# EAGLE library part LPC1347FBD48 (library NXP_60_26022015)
32-bit ARM Cortex-M3 microcontroller; up to 64 kB flash; up to 12 kB SRAM; USB device; USART; EEPROM The LPC1315/16/17/45/46/47 are ARM Cortex-M3 based microcontrollers for embedded applications featuring a high level of integration and low power consumption. The ARM Cortex-M3 is a next generation core that offers system enhancements such as enhanced debug features and a higher level of support block integration. The LPC1315/16/17/45/46/47 operate at CPU frequencies of up to 72 MHz. The ARM Cortex-M3 CPU incorporates a 3-stage pipeline and uses a Harvard architecture with separate local instruction and data buses as well as a third bus for peripherals. The ARM Cortex-M3 CPU also includes an internal prefetch unit that supports speculative branching. Equipped with a highly flexible and configurable Full-Speed USB 2.0 device controller available on the LPC1345/46/47, this series brings unparalleled design flexibility and seamless integration to today’s demanding connectivity solutions. The peripheral complement of the LPC1315/16/17/45/46/47 includes up to 64 kB of flash memory, 8 kB or 10 kB of SRAM data memory, one Fast-mode Plus I 2 C-bus interface, one RS-485/EIA-485 USART with support for synchronous mode and smart card interface, two SSP interfaces, four general purpose counter/timers, an 8-channel, 12-bit ADC, and up to 51 general purpose I/O pins. AAL Eindhoven MK
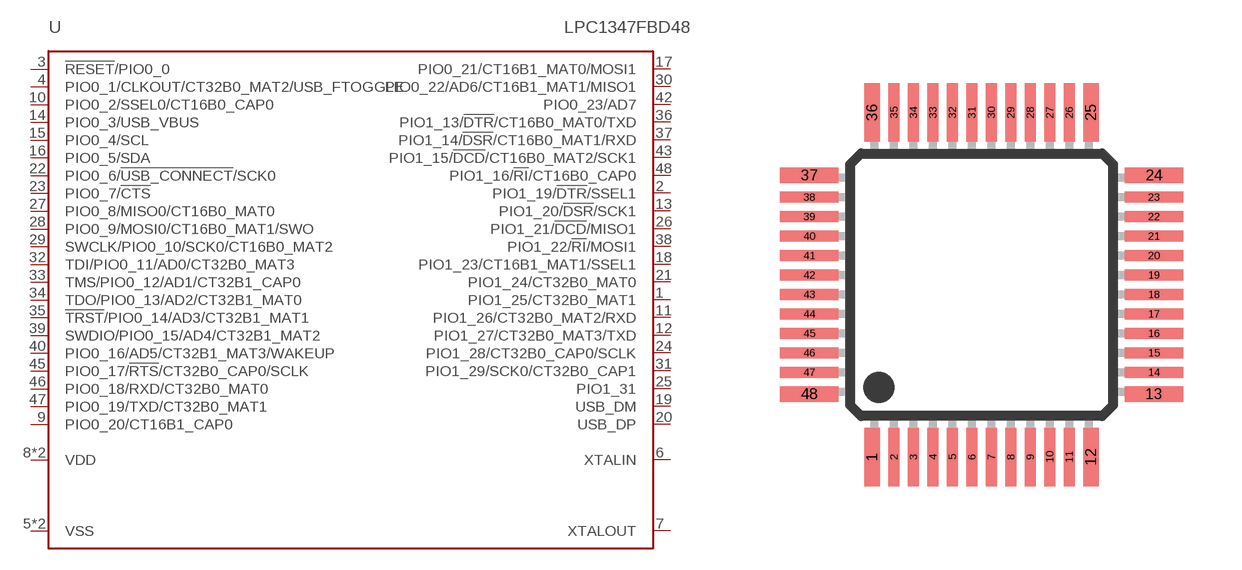
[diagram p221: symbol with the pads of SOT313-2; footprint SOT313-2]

Designator prefix U

## LPC1347FBD48 (EEPROM: 4kB; FLASH: 64kB; GPIO: 40; SRAM0: 8kB; SRAM1: 2kB; SRAM_USB: 2kB; USB: yes)  [SOT313-2]
1  PIO1_25/CT32B0_MAT1
2  PIO1_19/!DTR!/SSEL1
3  !RESET!/PIO0_0
4  PIO0_1/CLKOUT/CT32B0_MAT2/USB_FTOGGLE
5  VSS  pwr
6  XTALIN  in
7  XTALOUT  out
8  VDD  pwr
9  PIO0_20/CT16B1_CAP0
10  PIO0_2/SSEL0/CT16B0_CAP0
11  PIO1_26/CT32B0_MAT2/RXD
12  PIO1_27/CT32B0_MAT3/TXD
13  PIO1_20/!DSR!/SCK1
14  PIO0_3/USB_VBUS
15  PIO0_4/SCL
16  PIO0_5/SDA
17  PIO0_21/CT16B1_MAT0/MOSI1
18  PIO1_23/CT16B1_MAT1/SSEL1
19  USB_DM
20  USB_DP
21  PIO1_24/CT32B0_MAT0
22  PIO0_6/!USB_CONNECT!/SCK0
23  PIO0_7/!CTS!
24  PIO1_28/CT32B0_CAP0/SCLK
25  PIO1_31
26  PIO1_21/!DCD!/MISO1
27  PIO0_8/MISO0/CT16B0_MAT0
28  PIO0_9/MOSI0/CT16B0_MAT1/SWO
29  SWCLK/PIO0_10/SCK0/CT16B0_MAT2
30  PIO0_22/AD6/CT16B1_MAT1/MISO1
31  PIO1_29/SCK0/CT32B0_CAP1
32  TDI/PIO0_11/AD0/CT32B0_MAT3
33  TMS/PIO0_12/AD1/CT32B1_CAP0
34  TDO/PIO0_13/AD2/CT32B1_MAT0
35  !TRST!/PIO0_14/AD3/CT32B1_MAT1
36  PIO1_13/!DTR!/CT16B0_MAT0/TXD
37  PIO1_14/!DSR!/CT16B0_MAT1/RXD
38  PIO1_22/!RI!/MOSI1
39  SWDIO/PIO0_15/AD4/CT32B1_MAT2
40  PIO0_16/AD5/CT32B1_MAT3/WAKEUP
41  VSS  pwr
42  PIO0_23/AD7
43  PIO1_15/!DCD!/CT16B0_MAT2/SCK1
44  VDD  pwr
45  PIO0_17/!RTS!/CT32B0_CAP0/SCLK
46  PIO0_18/RXD/CT32B0_MAT0
47  PIO0_19/TXD/CT32B0_MAT1
48  PIO1_16/!RI!/CT16B0_CAP0

## Footprint SOT313-2 (pad centres in mm)
SOT313-2 LQFP48: plastic low profile quad flat package; 48 leads; body 7 x 7 x 1.4 mm JEDEC: MS-026 IEC: 136E05 Footprint according to NXP SOT313-2 specification, however the cornerpins are 0.4mm in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
smd 0.4 x 1.5: 1 -2.81,-4.425; 12 2.81,-4.425; 25 2.81,4.425; 36 -2.81,4.425
smd 0.28 x 1.5: 2 -2.25,-4.425; 3 -1.75,-4.425; 4 -1.25,-4.425; 5 -0.75,-4.425; 6 -0.25,-4.425; 7 0.25,-4.425; 8 0.75,-4.425; 9 1.25,-4.425; 10 1.75,-4.425; 11 2.25,-4.425; 26 2.25,4.425; 27 1.75,4.425; 28 1.25,4.425; 29 0.75,4.425; 30 0.25,4.425; 31 -0.25,4.425; 32 -0.75,4.425; 33 -1.25,4.425; 34 -1.75,4.425; 35 -2.25,4.425
smd 1.5 x 0.4: 13 4.425,-2.81; 24 4.425,2.81; 37 -4.425,2.81; 48 -4.425,-2.81
smd 1.5 x 0.28: 14 4.425,-2.25; 15 4.425,-1.75; 16 4.425,-1.25; 17 4.425,-0.75; 18 4.425,-0.25; 19 4.425,0.25; 20 4.425,0.75; 21 4.425,1.25; 22 4.425,1.75; 23 4.425,2.25; 38 -4.425,2.25; 39 -4.425,1.75; 40 -4.425,1.25; 41 -4.425,0.75; 42 -4.425,0.25; 43 -4.425,-0.25; 44 -4.425,-0.75; 45 -4.425,-1.25; 46 -4.425,-1.75; 47 -4.425,-2.25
